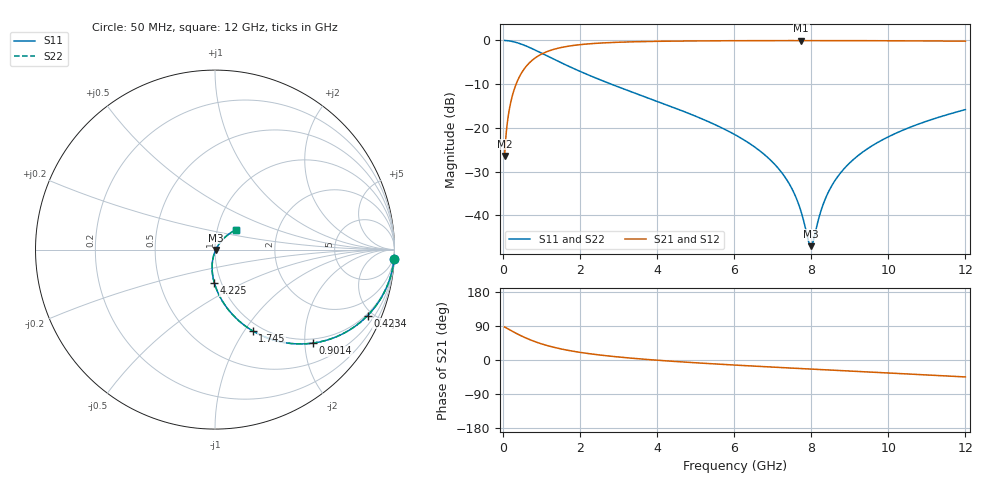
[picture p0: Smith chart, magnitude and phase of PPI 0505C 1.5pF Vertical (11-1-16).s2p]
# GHz S MA R 50
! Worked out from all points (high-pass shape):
!   1601 points, 50 MHz to 12 GHz, reference 50 ohm
!   highest |S21| = -0.04 dB at 7.743 GHz (marker M1); lowest = -26.4 dB at 50 MHz (marker M2)
!   |S21| within 3 dB of the highest: 1.026 GHz to end of sweep
!   lowest |S11| = -47.1 dB at 7.989 GHz (marker M3), VSWR 1.01, Z = 50.4 - j0.196 ohm
!   |S11| at or under -10 dB: 2.812 GHz to end of sweep
!   |S22| runs from -47.1 to 0.0 dB; largest |S21 - S12| = 0
!   S11 on the Smith chart (normalised r, x): 50 MHz: 1, -40; 423.4 MHz: 0.90, -4.67; 901.4 MHz: 0.90, -2.17; 1.745 GHz: 0.91, -1.09; 4.225 GHz: 0.93, -0.36; 12 GHz: 1.23, +0.28
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0.05  0.9989 -2.9  0.04777 87.1  0.04777 87.1  0.9989 -2.9
0.1470937  0.9902 -8.5  0.1393 81.5  0.1393 81.5  0.9902 -8.5
0.2068437  0.9809 -11.8  0.1942 78.2  0.1942 78.2  0.9809 -11.8
0.4234375  0.9263 -23.4  0.376 66.6  0.376 66.6  0.9263 -23.4
0.9014375  0.7534 -43.8  0.6562 46.1  0.6562 46.1  0.7534 -43.8
1.30475  0.6163 -55.8  0.7857 34.1  0.7857 34.1  0.6163 -55.8
1.745406  0.4984 -65.2  0.8648 24.6  0.8648 24.6  0.4984 -65.2
2.044156  0.4352 -70.1  0.8979 19.6  0.8979 19.6  0.4352 -70.1
4.038312  0.1986 -89.9  0.9767 -0.8  0.9767 -0.8  0.1986 -89.9
4.225031  0.1851 -91.2  0.9793 -2.2  0.9793 -2.2  0.1851 -91.2
6.025  0.08351 -100.8  0.9923 -13.4  0.9923 -13.4  0.08351 -100.8
7.145313  0.03453 -102.6  0.9948 -19.5  0.9948 -19.5  0.03453 -102.6
7.496344  0.02035 -99.3  0.9951 -21.4  0.9951 -21.4  0.02035 -99.3
7.742813  0.01088 -89.1  0.9951 -22.7  0.9951 -22.7  0.01088 -89.1
7.922063  0.005239 -56.2  0.9951 -23.6  0.9951 -23.6  0.005239 -56.2
7.989281  0.004438 -26.0  0.9951 -24.0  0.9951 -24.0  0.004438 -26.0
8.019156  0.004563 -11.1  0.995 -24.1  0.995 -24.1  0.004563 -11.1
8.332844  0.01414 45.5  0.9948 -25.7  0.9948 -25.7  0.01414 45.5
8.676406  0.02725 52.6  0.9944 -27.5  0.9944 -27.5  0.02725 52.6
9.229094  0.04868 53.9  0.9934 -30.3  0.9934 -30.3  0.04868 53.9
10.01331  0.07949 51.9  0.991 -34.3  0.991 -34.3  0.07949 51.9
12  0.1618 43.2  0.9801 -44.7  0.9801 -44.7  0.1618 43.2
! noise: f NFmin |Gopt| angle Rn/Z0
0.05  0.000954  0.9581  1.676  0.005127
1.372  0.005538  0.7566  5.874  0.004589
2.701  0.008674  0.702  9.503  0.005666
4.031  0.01144  0.6696  13.19  0.006568
5.36  0.01403  0.6477  16.87  0.007401
6.682  0.01654  0.6328  20.47  0.008214
8.012  0.01906  0.6228  24.03  0.009054
9.341  0.02163  0.6168  27.51  0.009946
10.67  0.02429  0.6143  30.92  0.01092
12  0.02708  0.6147  34.24  0.012
